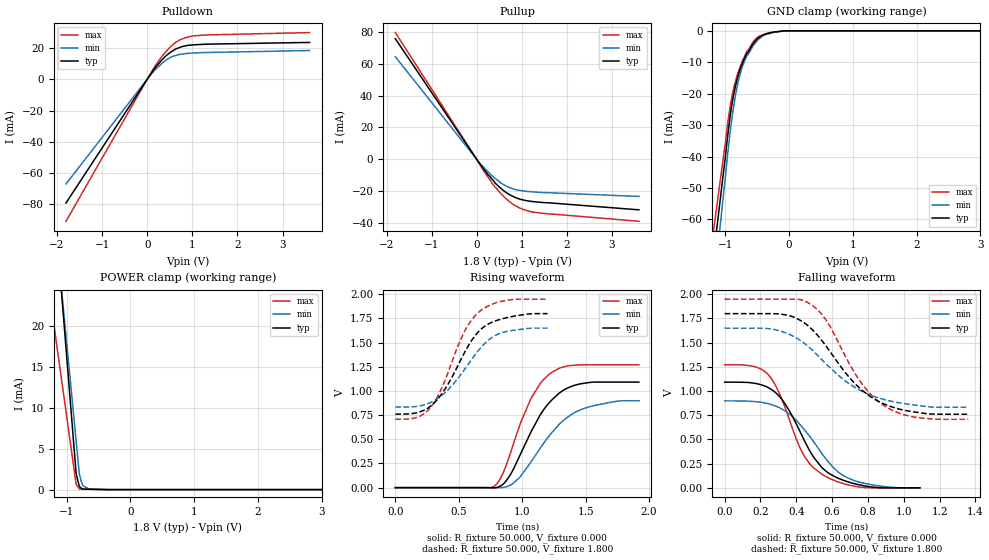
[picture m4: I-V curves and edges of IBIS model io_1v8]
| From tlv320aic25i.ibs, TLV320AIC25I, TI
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[Model]   io_1v8
Model_type I/O
Vinl=5.400E-01
Vinh=1.260E+00
Vref=0.000E+00
Rref=1.000E+06
Cref=2.000E-11
Vmeas=9.000E-01
C_comp   1.070E-12   1.070E-12   1.070E-12
[Voltage Range]   1.800E+00   1.650E+00   1.950E+00
[POWER Clamp Reference]   1.800E+00   1.650E+00   1.950E+00
[GND Clamp Reference]   0.000E+00   0.000E+00   0.000E+00
[Pullup Reference]   1.800E+00   1.650E+00   1.950E+00
[Pulldown Reference]   0.000E+00   0.000E+00   0.000E+00
[Temperature Range]   25   85   -40
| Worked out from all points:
|   slope of the pulldown table from 0 to 0.27 V, typ, clamps not added: 25.7 ohm
|   slope of the pullup table from 0 to 0.27 V, typ, clamps not added: 26.5 ohm
|   GND clamp passes 1 mA (typ) near -0.36 V on its own axis
|   POWER clamp passes 1 mA (typ) near -0.82 V on its own axis
|   rising waveform, R_fixture 50.000, V_fixture 0.000: 20-80 % time 269ps typ, 325ps min, 233ps max; typ from 0 V to 1.09 V
|   falling waveform, R_fixture 50.000, V_fixture 0.000: 20-80 % time 204ps typ, 236ps min, 178ps max; typ from 1.09 V to 0 V
|   rising waveform, R_fixture 50.000, V_fixture 1.800: 20-80 % time 276ps typ, 298ps min, 245ps max; typ from 0.761 V to 1.8 V
|   falling waveform, R_fixture 50.000, V_fixture 1.800: 20-80 % time 284ps typ, 319ps min, 245ps max; typ from 1.8 V to 0.761 V
[GND Clamp]
-1.8V     -177.3mA   -200.2mA   -157.4mA
-1.02V    -43.67mA   -50.61mA   -38.74mA
-960mV    -33.14mA   -38.86mA   -29.28mA
-900mV    -24.05mA   -28.52mA   -21.48mA
-840mV    -17.65mA   -20.61mA   -16.11mA
-800mV    -14.37mA   -16.57mA   -13.32mA
-740mV    -10.72mA   -11.95mA   -10.13mA
-660mV    -7.159mA   -7.876mA   -6.46mA
-480mV    -2.223mA   -2.767mA   -1.845mA
-360mV    -978.6uA   -1.135mA   -932uA
-40mV     0A         0A         0A
3.6V      0A         0A         0A
[POWER Clamp]
-1.8V     93.46mA    82.75mA    53.72mA
-1V       16.4mA     18.05mA    9.022mA
-850mV    1.946mA    5.92mA     641.4uA
-800mV    370.4uA    1.876mA    73.68uA
-750mV    60.36uA    504.1uA    65.92uA
-650mV    44.27uA    79.79uA    50.41uA
-375mV    0A         0A         7.756uA
3.6V      0A         0A         0A
[Pullup]
-1.81V    75.8mA     64.48mA    79.66mA
110mV     -4.437mA   -3.757mA   -5.106mA
330mV     -12.05mA   -10mA      -14.61mA
410mV     -14.92mA   -11.97mA   -17.54mA
550mV     -18.56mA   -15.16mA   -21.9mA
770mV     -22.8mA    -18.19mA   -27.51mA
1.03V     -25.52mA   -19.85mA   -31.48mA
1.27V     -26.65mA   -20.53mA   -33.25mA
3.61V     -31.73mA   -23.35mA   -38.98mA
[Pulldown]
-1.8V     -79.13mA   -67.01mA   -90.85mA
100mV     4.251mA    3.559mA    4.933mA
200mV     8.147mA    6.76mA     9.523mA
380mV     13.97mA    11.37mA    16.37mA
520mV     17.34mA    13.98mA    20.87mA
640mV     19.42mA    15.21mA    23.76mA
760mV     20.79mA    16.04mA    25.62mA
920mV     21.72mA    16.6mA     27.13mA
1.22V     22.28mA    17.04mA    28.16mA
3.6V      23.54mA    18.37mA    29.85mA
[Rising Waveform]
R_fixture = 50.000
V_fixture = 0.000
V_fixture_min = 0.000
V_fixture_max = 0.000
|  time   V(typ)   V(min)   V(max)
0s        0V         0V         0V
770ps     -2.092mV   0V         7.709mV
840ps     26.7mV     1.195mV    125mV
930ps     189mV      44.72mV    449.9mV
1.07ns    578.6mV    266.8mV    924.8mV
1.21ns    874.1mV    531.2mV    1.17V
1.33ns    1.012V     700.9mV    1.251V
1.46ns    1.074V     805.1mV    1.27V
1.74ns    1.092V     892.5mV    1.271V
1.92ns    1.092V     898.7mV    1.271V
[Falling Waveform]
R_fixture = 50.000
V_fixture = 0.000
V_fixture_min = 0.000
V_fixture_max = 0.000
|  time   V(typ)   V(min)   V(max)
0s        1.092V     898.7mV    1.271V
150ps     1.085V     893.8mV    1.259V
240ps     1.039V     870.9mV    1.176V
280ps     990.4mV    848mV      1.071V
330ps     886.8mV    802.2mV    865.2mV
440ps     507.8mV    612.1mV    343mV
540ps     215.7mV    361.8mV    144.5mV
630ps     103mV      169.9mV    63.78mV
720ps     45.22mV    77.94mV    18.82mV
1.09ns    0V         0V         0V
[Rising Waveform]
R_fixture = 50.000
V_fixture = 1.800
V_fixture_min = 1.650
V_fixture_max = 1.950
|  time   V(typ)   V(min)   V(max)
0s        760.7mV    833.7mV    707.4mV
170ps     775.1mV    840.7mV    727.3mV
280ps     844.5mV    881.8mV    833.6mV
370ps     977.7mV    958.3mV    1.041V
540ps     1.384V     1.212V     1.602V
600ps     1.52V      1.323V     1.732V
670ps     1.632V     1.443V     1.829V
750ps     1.704V     1.543V     1.891V
850ps     1.749V     1.607V     1.931V
1.2ns     1.8V       1.65V      1.95V
[Falling Waveform]
R_fixture = 50.000
V_fixture = 1.800
V_fixture_min = 1.650
V_fixture_max = 1.950
|  time   V(typ)   V(min)   V(max)
0s        1.8V       1.65V      1.95V
270ps     1.8V       1.639V     1.95V
380ps     1.768V     1.569V     1.95V
460ps     1.683V     1.471V     1.919V
570ps     1.455V     1.273V     1.723V
740ps     1.054V     1.024V     1.146V
810ps     947.7mV    961.3mV    977.5mV
880ps     875.1mV    917.7mV    862.2mV
1.06ns    783.8mV    855.8mV    731mV
1.36ns    760.7mV    833.7mV    707.4mV
[Ramp]
dV/dt_r   6.577E-01/2.685E-10   5.414E-01/3.230E-10   7.616E-01/2.297E-10
dV/dt_f   6.236E-01/2.836E-10   4.898E-01/3.185E-10   7.456E-01/2.438E-10
R_load = 50
